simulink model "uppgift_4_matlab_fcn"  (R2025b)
settings: Solver=VariableStepAuto  StartTime=0.0  StopTime=10.0  RelTol=1e-3
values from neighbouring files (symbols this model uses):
  AFs = 14.6    [Lektion_2.m]
  eta_vol = 0.8    [Lektion_2.m]
  m_dot_fi_start = m_dot_a_start/AFs    (= 0.000821917808219)    [Lektion_2.m]
  n_cyl = 4    [Lektion_2.m]
  N_init = 3000/60    (= 50)    [Lektion_2.m]
  n_r = 2    [Lektion_2.m]
  p_im_end = 70*1e3    (= 70000)    [Lektion_2.m]
  p_im_init = 40*1e3    (= 40000)    [Lektion_2.m]
  R = 280    [Lektion_2.m]
  T_i = 320    [Lektion_2.m]
  V_d = 0.55/1e3    (= 0.00055)    [Lektion_2.m]

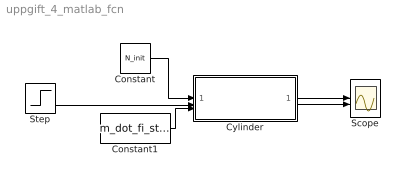
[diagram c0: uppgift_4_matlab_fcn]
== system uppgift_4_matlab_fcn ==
  Constant : Constant  Value=N_init
  Constant1 : Constant  Value=m_dot_fi_start
  Cylinder : Subsystem
  Scope : Scope  NumInputPorts=2
  Step : Step  Before=p_im_init  After=p_im_end  SampleTime=0
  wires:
  Constant/1 -> Cylinder/1(N [rps])
  Constant1/1 -> Cylinder/3(m_fi [kg/s])
  Step/1 -> Cylinder/2(p_im [Pa])
  Cylinder/1(m_ac [kg/s]) -> Scope/1
  Cylinder/2(lambda_c [-]) -> Scope/2

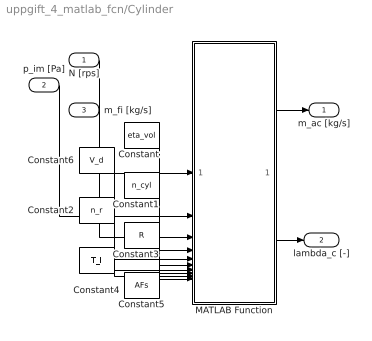
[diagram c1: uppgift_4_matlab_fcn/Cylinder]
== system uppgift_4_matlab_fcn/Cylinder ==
  N [rps] : Inport
  p_im [Pa] : Inport  Port=2
  m_fi [kg/s] : Inport  Port=3
  Constant : Constant  Value=eta_vol
  Constant1 : Constant  Value=n_cyl
  Constant2 : Constant  Value=n_r
  Constant3 : Constant  Value=R
  Constant4 : Constant  Value=T_i
  Constant5 : Constant  Value=AFs
  Constant6 : Constant  Value=V_d
  MATLAB Function : MATLAB Function  TreatAsAtomicUnit=on
  m_ac [kg/s] : Outport
  lambda_c [-] : Outport  Port=2
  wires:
  p_im [Pa]/1 -> MATLAB Function/2(p_im)
  m_fi [kg/s]/1 -> MATLAB Function/3(m_fi)
  MATLAB Function/2(lambda) -> lambda_c [-]/1
  MATLAB Function/1(m_ac) -> m_ac [kg/s]/1
  N [rps]/1 -> MATLAB Function/1(N)
  Constant/1 -> MATLAB Function/4(eta_vol)
  Constant5/1 -> MATLAB Function/10(AFs)
  Constant4/1 -> MATLAB Function/9(T)
  Constant3/1 -> MATLAB Function/8(R)
  Constant2/1 -> MATLAB Function/7(n_r)
  Constant1/1 -> MATLAB Function/6(n_cyl)
  Constant6/1 -> MATLAB Function/5(V_d)

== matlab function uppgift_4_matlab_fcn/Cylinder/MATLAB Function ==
function [m_ac, lambda]= fcn(N, p_im, m_fi,eta_vol,V_d,n_cyl,n_r,R,T,AFs)

m_ac = eta_vol*N*p_im*V_d*n_cyl/(n_r*R*T);

lambda = m_ac/m_fi * 1/AFs;
